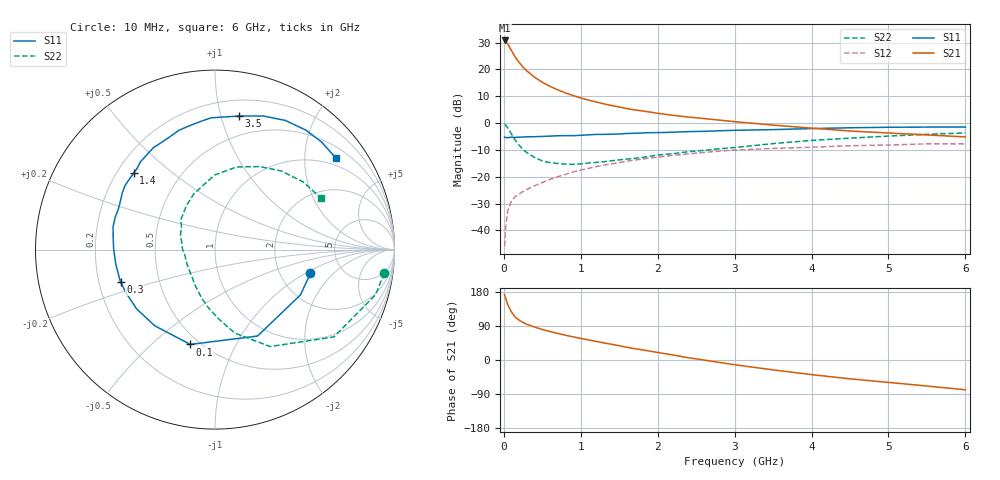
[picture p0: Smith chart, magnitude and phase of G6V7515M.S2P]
! SIEMENS Small Signal Semiconductors
! BFG193
! Si NPN RF Bipolar Junction Transistor in SOT223
! VCE = 0.75 V  IC = 15 mA
! Common Emitter S-Parameters:  August  1996
# GHz  S  MA  R  50
!  f  S11  S21  S12  S22
! GHz  MAG  ANG  MAG  ANG  MAG  ANG  MAG  ANG
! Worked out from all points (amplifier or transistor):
!   36 points, 10 MHz to 6 GHz, reference 50 ohm
!   highest |S21| = 30.8 dB at 10 MHz (marker M1)
!   |S21| within 3 dB of that: start of sweep to 83.76 MHz
!   unconditionally stable (mu >= 1): 697.3 MHz to 3.996 GHz
!   at 250 MHz: K = 0.69, MSG = 23.2 dB, |S12| = -25.5 dB
!   at 1.4 GHz: K = 1.08, MAG = 9.1 dB, |S12| = -15.2 dB
!   at 6 GHz: K = 0.98, MSG = 1.3 dB, |S12| = -7.7 dB
!   S11 on the Smith chart (normalised r, x): 10 MHz: 2.95, -1.12; 100 MHz: 0.45, -0.67; 300 MHz: 0.29, -0.15; 1.4 GHz: 0.27, +0.37; 3.5 GHz: 0.33, +1.14; 6 GHz: 0.78, +2.78
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0.01  0.548 -14.0  34.66 172.5  0.0051 87.4  0.9524 -7.9
0.02  0.5389 -27.9  33.78 165.9  0.0101 78.8  0.9293 -15.7
0.05  0.5368 -63.8  29.77 146.5  0.0232 66.4  0.8218 -36.3
0.1  0.546 -104.6  22.36 126.4  0.0361 53.7  0.6211 -60.4
0.15  0.5411 -128.3  16.81 113.0  0.043 48.8  0.4776 -76.7
0.2  0.5477 -142.8  13.44 105.0  0.0481 47.8  0.3862 -87.1
0.25  0.5506 -153.3  11.04 98.8  0.053 47.9  0.3219 -97.2
0.3  0.5568 -161.0  9.365 94.1  0.058 48.5  0.2824 -104.9
0.4  0.5589 -171.7  7.164 87.0  0.068 50.0  0.2283 -118.9
0.5  0.5647 179.6  5.761 80.5  0.0782 50.4  0.1978 -130.7
0.6  0.5718 173.0  4.842 75.2  0.0893 51.2  0.1839 -140.9
0.7  0.5821 167.3  4.174 70.1  0.1001 50.9  0.1768 -150.5
0.8  0.5846 162.1  3.649 65.5  0.1111 49.7  0.1727 -159.7
1.1  0.6048 148.8  2.687 53.0  0.1435 46.2  0.1807 179.3
1.4  0.6217 136.9  2.123 41.5  0.1739 40.8  0.1991 162.1
1.7  0.6474 127.1  1.761 29.9  0.2049 35.0  0.2207 148.2
2.2  0.6765 112.0  1.397 13.1  0.2508 23.6  0.2692 130.7
2.8  0.7192 96.2  1.138 -6.3  0.3009 9.7  0.3327 110.8
3.5  0.7565 79.7  0.918 -26.1  0.3383 -7.5  0.4154 90.3
4.5  0.8195 61.4  0.713 -49.7  0.379 -26.6  0.5254 61.7
5.5  0.8439 45.2  0.603 -68.7  0.4108 -48.5  0.6195 37.5
6  0.8447 37.2  0.553 -78.6  0.4101 -61.1  0.6565 25.9
